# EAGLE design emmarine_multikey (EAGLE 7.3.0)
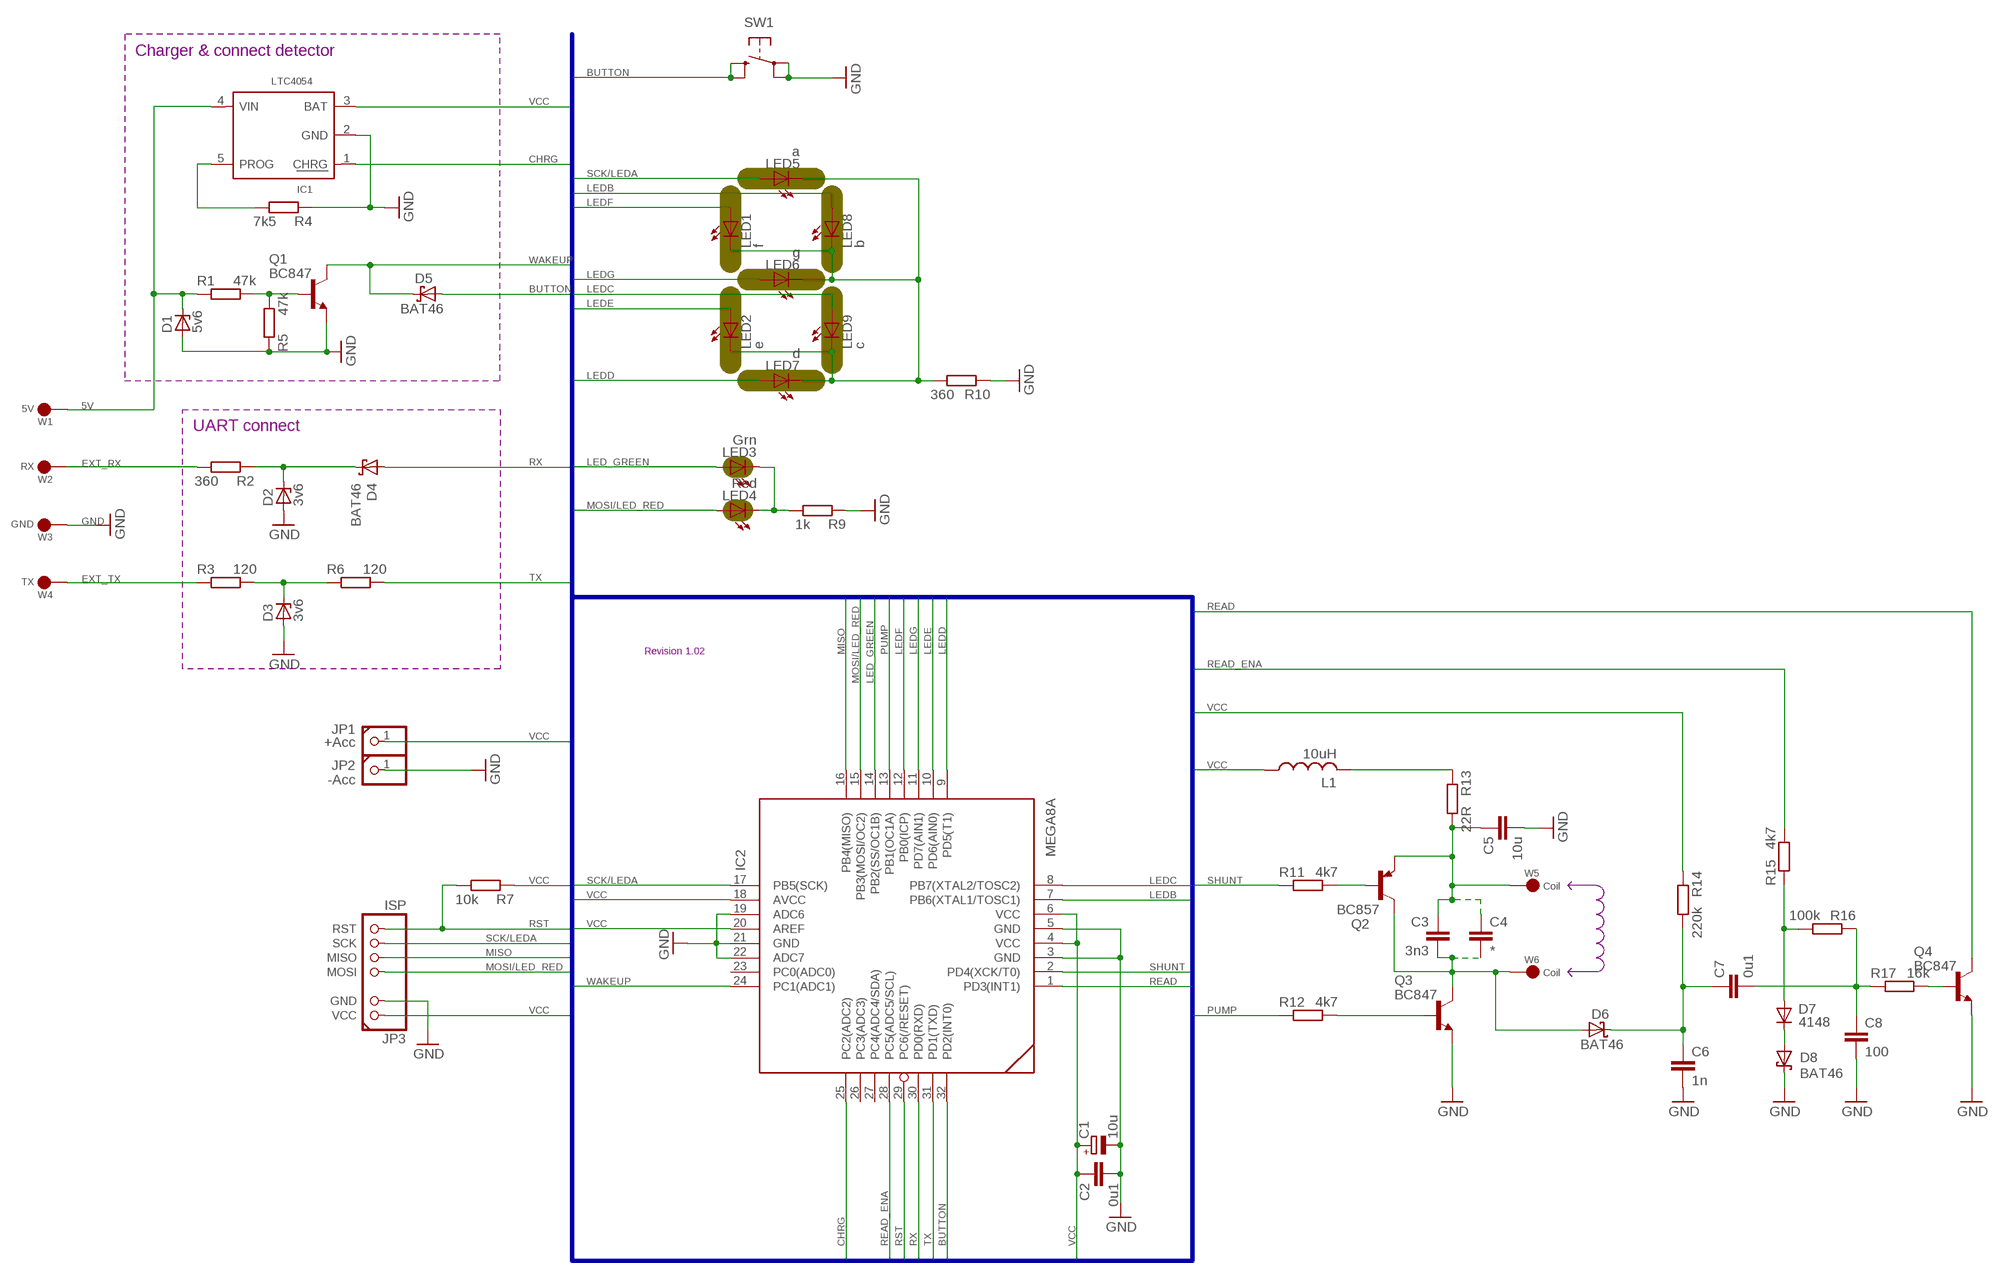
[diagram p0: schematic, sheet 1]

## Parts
C1  10u  CPOL-EUSMCA  [SMC_A]
C2  0u1  C-EUC0805T  [C0805T]
C3  3n3  C-EU050-025X075  [C050-025X075]
C4  *  C-EUC0805T  [C0805T]
C5  10u  C-EUC0805T  [C0805T]
C6  1n  C-EUC0805T  [C0805T]
C7  0u1  C-EUC0805T  [C0805T]
C8  100  C-EUC0805T  [C0805T]
D1  5v6  ZENER-DIODESOD80C  [SOD80C]
D2  3v6  ZENER-DIODESOD80C  [SOD80C]
D3  3v6  ZENER-DIODESOD80C  [SOD80C]
D4  BAT46  SCHOTTKY-DIODESOD80-R  [SOD80-R]
D5  BAT46  SCHOTTKY-DIODESOD80-R  [SOD80-R]
D6  BAT46  SCHOTTKY-DIODESOD80-R  [SOD80-R]
D7  4148  1N4148SMD  [SOD80-R]
D8  BAT46  SCHOTTKY-DIODESOD80-R  [SOD80-R]
IC1  LTC4054  [SOT23-5]
IC2  MEGA8A  MEGA8(TQFP)-AI  [TQFP32-08]
JP1  +Acc  CONN1X1/R  [1X01ROUND]
JP2  -Acc  CONN1X1/R  [1X01ROUND]
JP3  ISP  CONN1X7(2+4)_ISP+/P/NI  [1X07_ISP+POINTS_NO_INF]
L1  10uH  L-USL1210  [L1210]
LED1  f  LED0603  [CHIPLED_0603]
LED2  e  LED0603  [CHIPLED_0603]
LED3  Grn  LED0603  [CHIPLED_0603]
LED4  Red  LED0603  [CHIPLED_0603]
LED5  a  LED0603  [CHIPLED_0603]
LED6  g  LED0603  [CHIPLED_0603]
LED7  d  LED0603  [CHIPLED_0603]
LED8  b  LED0603  [CHIPLED_0603]
LED9  c  LED0603  [CHIPLED_0603]
Q1  BC847  [SOT23_THIN]
Q2  BC857  [SOT23_THIN]
Q3  BC847  [SOT23_THIN]
Q4  BC847  [SOT23_THIN]
R1  47k  R-EU_R0805T  [R0805T]
R2  360  R-EU_R0805T  [R0805T]
R3  120  R-EU_R0805T  [R0805T]
R4  7k5  R-EU_R0805T  [R0805T]
R5  47k  R-EU_R0805T  [R0805T]
R6  120  R-EU_R0805T  [R0805T]
R7  10k  R-EU_R0805T  [R0805T]
R9  1k  R-EU_R0805T  [R0805T]
R10  360  R-EU_R0805T  [R0805T]
R11  4k7  R-EU_R0805T  [R0805T]
R12  4k7  R-EU_R0805T  [R0805T]
R13  22R  R-EU_R0805T  [R0805T]
R14  220k  R-EU_R0805T  [R0805T]
R15  4k7  R-EU_R0805T  [R0805T]
R16  100k  R-EU_R0805T  [R0805T]
R17  16k  R-EU_R0805T  [R0805T]
SW1  TACT_BUTTON24.2X3.5  [BUTTON_SMD_4.2X3.5]
W1  5V  SIMPLE_WIRE/R2  [SIMPLE_WIRE_R2]
W2  RX  SIMPLE_WIRE/R2  [SIMPLE_WIRE_R2]
W3  GND  SIMPLE_WIRE/R2  [SIMPLE_WIRE_R2]
W4  TX  SIMPLE_WIRE/R2  [SIMPLE_WIRE_R2]
W5  Coil  SIMPLE_WIRE/R  [SIMPLE_WIRE_R]
W6  Coil  SIMPLE_WIRE/R  [SIMPLE_WIRE_R]

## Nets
5V: D1.C IC1.4(VIN) R1.1 W1.WIRE
BUTTON: D5.A IC2.32(PD2(INT0)) SW1.S SW1.S@1(S)
CHRG: IC1.1(CHRG) IC2.25(PC2(ADC2))
COIL: C3.2 C4.2 D6.A Q2.3(C) Q3.3(C) W6.WIRE
EXT_RX: R2.2 W2.WIRE
EXT_TX: R3.1 W4.WIRE
GND: C1.- C2.2 C5.2 C6.2 C8.2 D1.A D2.A D3.A D8.C IC1.2(GND) IC2.3(GND) IC2.5(GND) IC2.19(ADC6) IC2.21(GND) IC2.22(ADC7) JP2.1 JP3.GND Q1.2(E) Q3.2(E) Q4.2(E) R4.1 R5.1 R9.1 R10.1 SW1.P SW1.P@1(P) W3.WIRE
LED_GREEN: IC2.14(PB2(SS/OC1B)) LED3.A
LEDB: IC2.7(PB6(XTAL1/TOSC1)) LED8.A
LEDC: IC2.8(PB7(XTAL2/TOSC2)) LED9.A
LEDD: IC2.9(PD5(T1)) LED7.A
LEDE: IC2.10(PD6(AIN0)) LED2.A
LEDF: IC2.12(PB0(ICP)) LED1.A
LEDG: IC2.11(PD7(AIN1)) LED6.A
MISO: IC2.16(PB4(MISO)) JP3.MISO
MOSI/LED_RED: IC2.15(PB3(MOSI/OC2)) JP3.MOSI LED4.A
N$1: C6.1 C7.1 D6.C R14.2
N$2: D3.C R3.2 R6.1
N$3: Q2.1(B) R11.2
N$4: Q3.1(B) R12.2
N$5: Q1.1(B) R1.2 R5.2
N$6: D2.C D4.C R2.1
N$7: LED1.C LED2.C LED5.C LED6.C LED7.C LED8.C LED9.C R10.2
N$9: L1.2 R13.1
N$10: LED3.C LED4.C R9.2
N$11: C3.1 C4.1 C5.1 Q2.2(E) R13.2 W5.WIRE
N$12: IC1.5(PROG) R4.2
N$15: Q4.1(B) R17.2
N$16: C7.2 C8.1 R16.1 R17.1
N$17: D7.A R15.1 R16.2
N$18: D7.C D8.A
PUMP: IC2.13(PB1(OC1A)) R12.1
READ: IC2.1(PD3(INT1)) Q4.3(C)
READ_ENA: IC2.28(PC5(ADC5/SCL)) R15.2
RST: IC2.29(PC6(/RESET)) JP3.RST R7.2
RX: D4.A IC2.30(PD0(RXD))
SCK/LEDA: IC2.17(PB5(SCK)) JP3.SCK LED5.A
SHUNT: IC2.2(PD4(XCK/T0)) R11.1
TX: IC2.31(PD1(TXD)) R6.2
VCC: C1.+ C2.1 IC1.3(BAT) IC2.4(VCC) IC2.6(VCC) IC2.18(AVCC) IC2.20(AREF) JP1.1 JP3.+5V(VCC) L1.1 R7.1 R14.1
WAKEUP: D5.C IC2.24(PC1(ADC1)) Q1.3(C)
Unconnected: IC2.23(PC0(ADC0)) IC2.26(PC3(ADC3)) IC2.27(PC4(ADC4/SDA))

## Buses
VCC,MOSI/LED_RED,MISO,SCK/LEDA,RST,RX,RX_UP,TX,PUMP,SHUNT,READ,READ_ENA,LEDB,LEDC,LEDD,LEDE,LEDF,LEDG,LED_GREEN,BUTTON,WAKEUP,CHRG

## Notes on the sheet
- Charger & connect detector
- UART connect
- Revision 1.02

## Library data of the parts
C1 = rcl:CPOL-EU: POLARIZED CAPACITOR, European symbol
C2-C8 = rcl:C-EU: CAPACITOR, European symbol
D1-D3 = diode:ZENER-DIODE: Z-Diode
D4-D6 D8 = diode:SCHOTTKY-DIODE: Schottky Diode
D7 = diode:1N4148: DIODE
IC1 = v-reg-AL:LTC4054
IC2 = atmel:MEGA8(TQFP): MICROCONTROLLER 8 Kbytes FLASH, 1 kbytes SRAM, 512 bytes EEPROM, USART, 6-channel 10 bit ADC, 2-channel 8 bit ADC Pin compatible with Atmega48, ATMega88, ATMega168 Source: avr.lbr; MPN: ATMEGA8-16AU; OC_FARNELL: 9171371; OC_NEWARK: 73M8863
JP1 JP2 = pinhead-AL:CONN1X1
JP3 = pinhead-AL:CONN1X7(2+4)_ISP+: PIN HEADER
L1 = rcl:L-US: INDUCTOR, American symbol
LED1-LED9 = led-AL:LED
Q1 Q3 Q4 = transistor-npn-AL:BC847*: NPN Transistor
Q2 = transistor-pnp-AL:BC857*: PNP Transistror
R1-R7 R9-R17 = rcl:R-EU_: RESISTOR, European symbol
SW1 = switch-misc-AL:TACT_BUTTON2
W1-W6 = connectors-AL:SIMPLE_WIRE

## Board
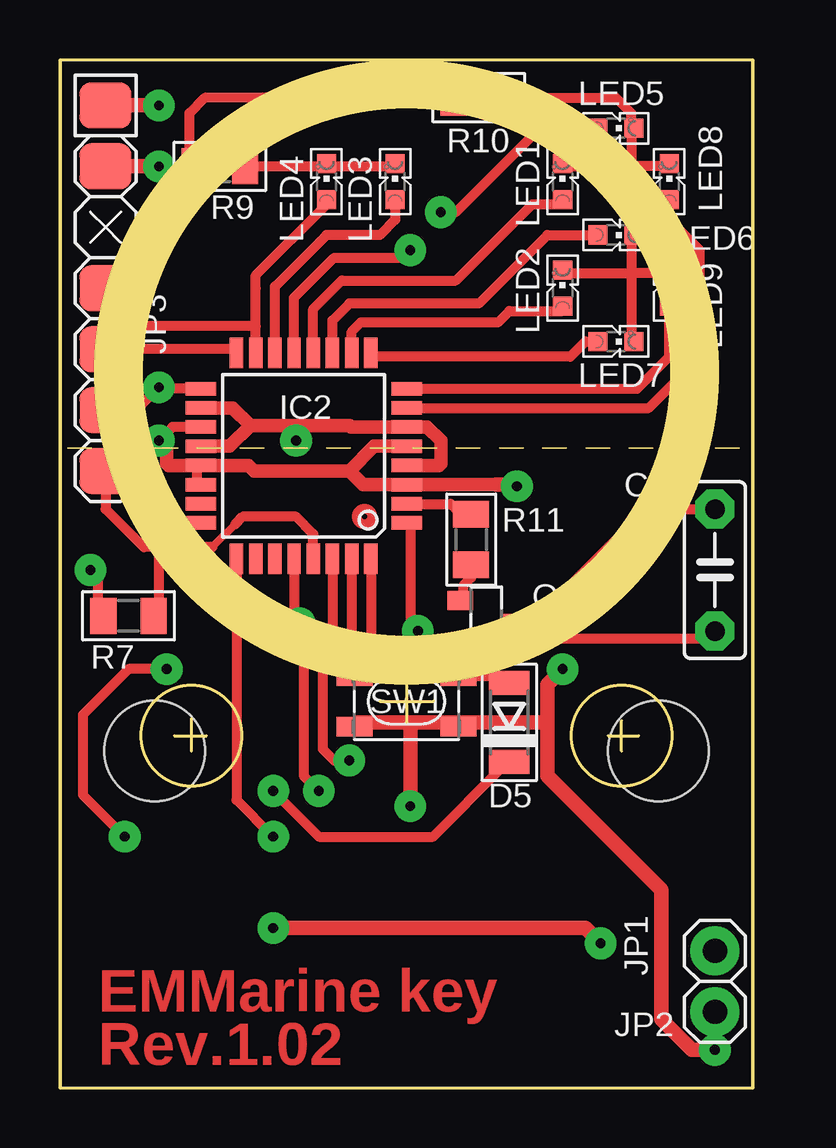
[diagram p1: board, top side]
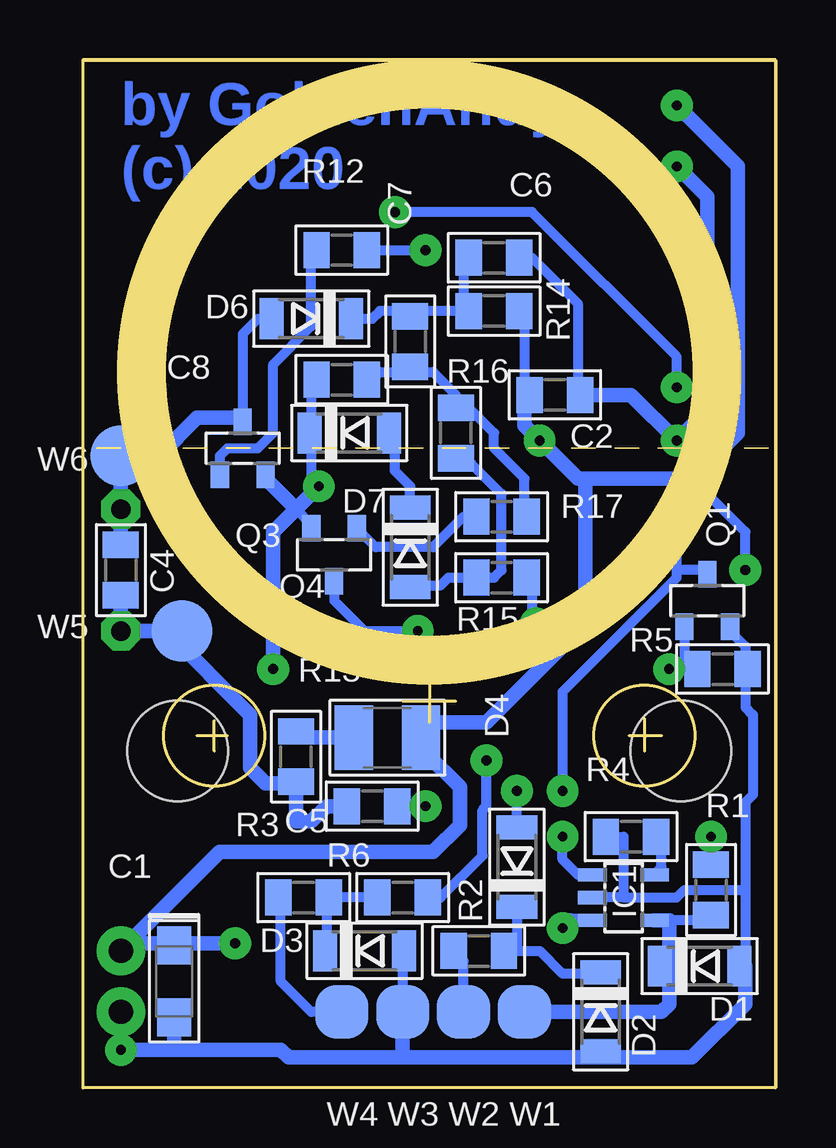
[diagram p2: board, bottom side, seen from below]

Size 28.88 x 42.85 mm. Coordinates in mm from the lower left corner, seen from the top.
Outline: 0,0 28.88,0 28.88,42.85 0,42.85 0,0
Copper layers (1*16): Top 0.035mm / dielectric 1.5mm / Bottom 0.035mm
Design rules "default": minimum track width 12mil, minimum drill 14mil, track to track 8mil, track to pad 8mil, pad to pad 8mil, via to via 8mil, smd to smd 8mil, copper to edge 20mil, drill to drill 30mil, minimum pad ring 16mil, minimum via ring 18mil, stop-mask expansion 4mil, vias tented up to drill 0mil, thermal gap 16mil
Holes 4.19 mm at 3.95,14.05 24.94,14.05
Milling: area 3.4,12.6 to 7.6,16.8; area 21.3,12.6 to 25.5,16.8; area 2.4,17.8 to 26.4,41.8; 26 lines

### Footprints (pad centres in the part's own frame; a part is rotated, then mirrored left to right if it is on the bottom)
SMC_A = smd 1.6 x 1.4: + -1.5,0; - 1.5,0
C0805T = smd 1.1 x 1.5: 1 -1.05,0; 2 1.05,0
C050-025X075 = drill 0.813 octagon: 1 -2.54,0; 2 2.54,0
SOD80C = smd 1 x 1.7: A 1.65,0; C -1.65,0
SOD80-R = smd 1 x 1.7: A 1.65,0; C -1.65,0
SOT23-5 = smd 0.55 x 1.2: 1 -0.95,-1.3; 2 0,-1.3; 3 0.95,-1.3; 4 0.95,1.3; 5 -0.95,1.3
TQFP32-08 = smd 1.27 x 0.559: 1 -4.293,2.8; 2 -4.293,2; 3 -4.293,1.2; 4 -4.293,0.4; 5 -4.293,-0.4; 6 -4.293,-1.2; 7 -4.293,-2; 8 -4.293,-2.8; 17 4.293,-2.8; 18 4.293,-2; 19 4.293,-1.2; 20 4.293,-0.4; 21 4.293,0.4; 22 4.293,1.2; 23 4.293,2; 24 4.293,2.8 | smd 0.559 x 1.27: 9 -2.8,-4.293; 10 -2,-4.293; 11 -1.2,-4.293; 12 -0.4,-4.293; 13 0.4,-4.293; 14 1.2,-4.293; 15 2,-4.293; 16 2.8,-4.293; 25 2.8,4.293; 26 2,4.293; 27 1.2,4.293; 28 0.4,4.293; 29 -0.4,4.293; 30 -1.2,4.293; 31 -2,4.293; 32 -2.8,4.293
1X01ROUND = drill 1.016 pad 2.032: 1 0,0
1X07_ISP+POINTS_NO_INF = smd 1.905 x 2.159: +5V -7.62,0; GND -5.08,0; MISO 2.54,0; MOSI 0,0; RST 7.62,0; SCK 5.08,0
L1210 = smd 1.6 x 2.7: 1 -1.4,0; 2 1.4,0
CHIPLED_0603 = smd 0.8 x 0.8: A 0,-0.75; C 0,0.75
SOT23_THIN = smd 0.8 x 1.1: 1 -0.95,-1.1; 2 0.95,-1.1; 3 0,1.1
R0805T = smd 1.1 x 1.5: 1 -1.05,0; 2 1.05,0
BUTTON_SMD_4.2X3.5 = smd 1.5 x 0.8: P -2.17,1.055; P@1 2.17,1.055; S -2.17,-1.055; S@1 2.17,-1.055
SIMPLE_WIRE_R2 = smd 2.223 x 2.223: WIRE 0,0
SIMPLE_WIRE_R = smd 2.54 x 2.54: WIRE 0,0

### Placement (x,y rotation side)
C1  25.08,4.45 270 bottom
C2  9.21,28.89 0 bottom
C3  27.3,21.59 90 top
C4  27.3,21.59 90 bottom
C5  16.83,11.75 0 bottom
C6  11.75,34.61 0 bottom
C7  15.24,31.12 270 bottom
C8  18.1,29.53 180 bottom
D1  3.18,5.08 0 bottom
D2  7.3,3.18 270 bottom
D3  17.15,5.71 0 bottom
D4  10.8,9.21 90 bottom
D5  18.73,15.24 90 top
D6  19.37,32.07 180 bottom
D7  15.24,22.54 270 bottom
D8  17.78,27.3 0 bottom
IC1  6.35,7.94 270 bottom
IC2  10.16,26.35 180 top
JP1  27.3,5.71 0 top
JP2  27.3,3.18 0 top
JP3  1.91,33.34 270 top
L1  16.19,14.61 180 bottom
LED1  20.95,37.78 0 top
LED2  20.95,33.34 0 top
LED3  13.97,37.78 0 top
LED4  11.11,37.78 0 top
LED5  23.18,40.01 270 top
LED6  23.18,35.56 270 top
LED7  23.18,31.12 270 top
LED8  25.4,37.78 0 top
LED9  25.4,33.34 0 top
Q1  2.86,20.32 0 bottom
Q2  17.78,19.37 270 top
Q3  22.23,26.67 0 bottom
Q4  18.41,22.23 180 bottom
R1  2.7,8.26 90 bottom
R2  12.38,5.71 180 bottom
R3  19.69,7.94 0 bottom
R4  6.03,10.48 0 bottom
R5  2.22,17.46 180 bottom
R6  15.56,7.94 0 bottom
R7  2.86,19.69 0 top
R9  6.67,38.42 0 top
R10  17.46,41.27 0 top
R11  17.15,22.86 270 top
R12  18.1,34.93 180 bottom
R13  20,13.81 270 bottom
R14  11.75,32.38 180 bottom
R15  11.43,21.27 0 bottom
R16  13.34,27.3 270 bottom
R17  11.43,23.81 180 bottom
SW1  14.45,16.11 180 top
W1  10.48,3.18 0 bottom
W2  13.02,3.18 0 bottom
W3  15.56,3.18 0 bottom
W4  18.1,3.18 0 bottom
W5  24.77,19.05 0 bottom
W6  27.3,26.35 0 bottom

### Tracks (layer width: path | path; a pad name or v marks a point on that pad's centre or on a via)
5V
  Bottom 0.406: R1.1 2.54,6.98 IC1.4
  Bottom 0.61: W1.WIRE 4.76,3.18 4.45,3.49 4.45,5.4 | IC1.4 4.76,6.99 | 4.76,6.99 5.08,6.98 | 4.76,6.99 4.45,6.98 4.45,5.4 | D1.C 4.45,5.4
BUTTON
  Top 0.406: IC2.32 12.96,17.41 12.7,17.15 12.68,17.17 SW1.S@1 SW1.S 16.64,17.15 18.73,17.15 D5.A
CHRG  (via drill 0.41)
  Top 0.406: v8.89,10.48 7.36,12.01 IC2.25
  Bottom 0.406: IC1.1 8.25,8.89 8.89,9.52 v8.89,10.48
COIL
  Top 0.406: Q2.3 19.69,19.37 24.45,24.13 C3.2
  Bottom 0.406: Q3.3 22.23,31.43 21.59,32.07 D6.A
  Bottom 0.61: C4.2 C3.2 W6.WIRE 25.72,26.35 24.13,27.94 22.23,27.94 Q3.3
EXT_RX
  Bottom 0.406: W2.WIRE 13.02,5.3 R2.2
EXT_TX
  Bottom 0.406: W4.WIRE 19.37,3.18 20.64,4.45 20.64,7.84 R3.1
GND  (via drill 0.41)
  Top 0.406: IC2.22 5.79,25.15 5.71,25.08 5.71,25.8 IC2.21 | 4.45,26.99 4.45,27.3 4.69,27.55 IC2.19 | 20,15.24 20.32,15.24 | SW1.P@1 12.28,15.13 12.38,15.24 | SW1.P 16.65,15.06 16.83,15.24 | R10.1 6.03,41.27 5.4,40.64 5.4,38.42 | v4.13,38.42 5.4,38.42 | R9.1 5.4,38.42
  Top 0.559: IC2.5 13.1,26.75 12.07,25.72 | 12.07,25.72 8.09,25.72 7.86,25.95 IC2.21 4.53,25.95 4.45,26.04 4.45,26.99 v4.13,26.99 | 12.07,25.72 12.63,25.15 IC2.3 18.17,25.15
  Top 0.61: JP3.GND v4.13,38.42 | v20.95,17.46 20.32,16.83 20.32,15.24 20.32,13.02 25.08,8.26 25.08,2.86 26.35,1.59 v27.3,1.59 | v14.61,11.75 14.61,15.24 | 12.38,15.24 14.61,15.24 | 14.61,15.24 16.83,15.24 20,15.24 | 18.17,25.15 18.8,25.15 v19.05,25.08
  Bottom 0.406: C6.2 10.16,34.61 8.26,32.7 8.26,28.67 C2.2 | Q4.2 19.37,23.49 20,24.13 | v19.05,25.08 19.37,25.4 19.37,27.3 D8.C 19.37,27.37 19.37,29.53 C8.2 | D3.A 15.56,5.71 W3.WIRE | 1.27,17.46 1.27,18.41 1.91,19.05 Q1.2 | 1.27,17.46 1.27,15.88 0.95,15.56 0.95,12.22 1.27,11.91 1.27,8.26 | 1.27,8.26 1.27,5.08 D1.A | R4.1 6.35,10.48 6.35,7.94 | 6.35,7.94 IC1.2 | 6.35,7.94 4.13,7.94 3.81,8.26 1.27,8.26 | R5.1 1.27,17.46
  Bottom 0.61: v4.13,38.42 2.86,37.15 2.86,28.26 v4.13,26.99 6.03,28.89 C2.2 | v19.05,25.08 20,24.13 | 20,24.13 20.95,23.18 v20.95,17.46 | JP2.1 v27.3,1.59 25.08,1.59 | Q3.2 21.27,25.4 20,24.13 | C5.2 v14.61,11.75 | C1.- 25.08,1.59 | 25.08,1.59 20.64,1.59 20.32,1.27 15.56,1.27 | 15.56,1.27 W3.WIRE | D2.A 7.3,1.27 | 7.3,1.27 15.56,1.27 | 1.27,5.08 1.27,3.49 3.49,1.27 7.3,1.27
LED_GREEN
  Top 0.406: IC2.14 8.96,33.41 11.11,35.56 13.34,35.56 13.97,36.2 LED3.A
LEDB
  Top 0.406: IC2.7 24.54,28.35 26.67,30.48 26.67,34.93 25.4,36.2 LED8.A
LEDC
  Top 0.406: IC2.8 24.07,29.15 25.4,30.48 LED9.A
LEDD
  Top 0.406: IC2.9 13.12,30.48 21.27,30.48 21.91,31.12 LED7.A
LEDE
  Top 0.406: IC2.10 12.16,31.53 12.54,31.91 18.26,31.91 18.73,32.38 20.95,32.38 LED2.A
LEDF
  Top 0.406: IC2.12 10.56,32.47 11.75,33.66 16.51,33.66 19.69,36.83 20.95,36.83 LED1.A
LEDG
  Top 0.406: IC2.11 11.36,32 12.07,32.7 17.46,32.7 20.32,35.56 LED6.A
MISO
  Top 0.406: IC2.16 7.36,30.74 7.3,30.8 JP3.MISO
MOSI/LED_RED
  Top 0.406: 8.16,31.75 3.49,31.75 JP3.MOSI | IC2.15 8.16,31.75 | LED4.A 11.11,36.83 8.16,33.88 8.16,33.34 8.16,31.75
N$1
  Bottom 0.406: C6.1 13.02,34.61 13.02,32.38 R14.2 15.24,32.38 | 15.24,32.38 16.51,32.38 16.83,32.07 D6.C | C7.1 15.24,32.38
N$2
  Bottom 0.406: R6.1 R3.2 18.73,7.94 18.73,5.78 D3.C
N$3
  Top 0.406: R11.2 17.15,21.27 16.83,20.95 16.83,20.32 Q2.1
N$4
  Bottom 0.406: Q3.1 23.18,26.36 22.86,26.67 21.59,26.67 20.95,27.3 20.95,30.16 19.37,31.75 19.37,34.93 R12.2
N$5  (via drill 0.41)
  Top 0.406: v4.45,17.46 2.86,17.46 0.95,15.56 0.95,12.22 v2.7,10.48
  Bottom 0.406: Q1.1 3.81,19.05 3.81,17.46 | 3.81,17.46 3.49,17.46 3.27,17.37 R5.2 | 3.81,17.46 v4.45,17.46 | v2.7,10.48 R1.2
N$6
  Bottom 0.406: R2.1 10.8,5.71 | D4.C 10.8,5.71 | 10.8,5.71 9.84,5.71 8.89,4.76 7.3,4.76 D2.C
N$7
  Top 0.406: R10.2 23.18,41.27 23.81,40.64 23.81,40.01 | LED5.C 23.81,40.01 | 23.81,40.01 23.81,38.42 | 23.81,38.42 23.81,35.56 | 23.81,35.56 23.81,33.97 | 23.81,33.97 23.81,31.12 LED7.C | LED6.C 23.81,35.56 | LED2.C 20.95,33.97 23.81,33.97 | LED9.C 25.4,33.97 23.81,33.97 | LED8.C 25.4,38.42 23.81,38.42 | LED1.C 20.95,38.42 23.81,38.42
N$9
  Bottom 0.406: 19.91,14.61 R13.1
  Bottom 0.61: L1.2 19.91,14.61
N$10
  Top 0.406: R9.2 11.11,38.42 | 11.11,38.42 13.97,38.42 LED3.C | LED4.C 11.11,38.42
N$11
  Top 0.406: Q2.2 16.83,18.42 16.83,18.41 17.62,18.41 17.78,18.26 19.84,18.26 20.32,18.73 26.99,18.73 C3.1
  Bottom 0.61: C5.1 18.73,11.75 19.37,11.11 20,11.11 R13.2 20.06,12.7 21.27,12.7 21.91,13.34 21.91,15.56 25.4,19.05 | W5.WIRE 25.4,19.05 | 25.4,19.05 C3.1 C4.1
N$12
  Bottom 0.406: IC1.5 4.77,9.2 4.76,9.52 4.76,10.48 R4.2
N$15
  Bottom 0.406: R17.2 13.02,23.81 14.29,22.54 16.68,22.54 Q4.1
N$16
  Bottom 0.406: R17.1 10.48,23.81 10.48,25.4 11.75,26.67 11.75,27.3 12.7,28.26 13.24,28.26 R16.1 13.34,28.89 14.29,29.84 15.24,29.84 C7.2 15.46,29.84 16.51,29.84 16.83,29.53 C8.1
N$17
  Bottom 0.406: R16.2 13.34,26.04 12.7,26.04 11.43,24.77 11.43,21.59 11.75,21.27 R15.1 13.65,21.27 13.97,20.95 15.24,20.95 D7.A
N$18
  Bottom 0.406: D7.C 15.24,25.08 15.88,25.72 15.88,27.3 D8.A
PUMP  (via drill 0.41)
  Top 0.406: IC2.13 9.76,32.94 11.43,34.61 14.29,34.61 v14.61,34.93
  Bottom 0.406: R12.1 v14.61,34.93
READ  (via drill 0.41)
  Top 0.406: IC2.1 14.55,23.55 14.61,23.5 14.61,19.37 v14.92,19.05
  Bottom 0.406: Q4.3 18.41,20.32 17.15,19.05 v14.92,19.05
READ_ENA  (via drill 0.41)
  Top 0.406: IC2.28 9.76,19.61 v10,19.37
  Bottom 0.406: R15.2 10.16,21.27 10.16,19.53 v10,19.37
RST
  Top 0.305: 7.3,23.5 6.35,22.54
  Top 0.406: IC2.29 10.56,23.09 9.84,23.81 7.62,23.81 7.3,23.5 | 6.35,22.54 4.13,22.54 | 4.13,22.54 3.49,22.54 1.91,24.13 JP3.RST | R7.2 4.13,19.69 4.13,22.54
RX  (via drill 0.41)
  Top 0.406: IC2.30 11.36,19.06 10.16,17.86 10.16,13.02 v10.8,12.38
  Bottom 0.406: D4.A v10.8,12.38
SCK/LEDA  (via drill 0.41)
  Top 0.406: IC2.17 4.19,29.15 v4.13,29.21 3.18,28.26 JP3.SCK | v15.88,36.51 16.51,36.51 20,40.01 LED5.A
  Bottom 0.406: v4.13,29.21 4.13,30.48 10.16,36.51 v15.88,36.51
SHUNT
  Top 0.406: R11.1 17.15,24.13 16.51,24.13 16.29,24.35 IC2.2
TX  (via drill 0.41)
  Top 0.406: IC2.31 12.16,18.91 10.95,17.7 10.95,14.13 11.43,13.65 v12.07,13.65
  Bottom 0.406: R6.2 13.97,7.94 12.22,9.68 12.22,11.59 12.07,11.75 v12.07,13.65
VCC  (via drill 0.41)
  Top 0.406: R7.1 1.59,19.69 1.59,21.27 v1.27,21.59
  Top 0.559: IC2.4 15.79,25.95 15.88,26.04 15.88,26.99 15.31,27.55 IC2.6 12.13,27.55 12.07,27.62 9.84,27.62 | IC2.20 7.07,26.75 7.94,27.62 | IC2.18 7.21,28.35 7.94,27.62 | 7.94,27.62 9.84,27.62 | v9.84,26.99 9.84,27.62
  Top 0.61: JP3.+5V v4.13,40.96 | v8.89,6.67 21.91,6.67 v22.54,6.03
  Bottom 0.406: C2.1 10.48,28.58 | R14.1 10.48,32.38 10.48,27.94 | v1.27,21.59 1.27,23.18 3.49,25.4
  Bottom 0.559: IC1.3 7.94,6.99 8.57,6.98
  Bottom 0.61: v4.13,40.96 1.59,38.42 1.59,27.3 3.49,25.4 7.94,25.4 | 7.94,25.4 8.26,25.4 v9.84,26.99 10.48,27.62 10.48,27.94 10.48,28.58 | 14.61,14.61 L1.1 | 14.61,14.61 14.61,13.97 13.18,12.54 13.18,10.95 14.29,9.84 23.18,9.84 JP1.1 26.99,6.03 25.08,6.03 C1.+ 25,6.03 v22.54,6.03 | 14.61,14.61 14.61,15.24 12.07,15.24 7.94,19.37 7.94,25.4 | 8.57,6.98 v8.89,6.67
WAKEUP  (via drill 0.41)
  Top 0.406: IC2.24 4.39,23.55 v4.13,23.81 | v8.89,12.38 10.8,10.48 15.56,10.48 18.41,13.34 18.73,13.34 D5.C
  Bottom 0.406: v8.89,12.38 8.89,16.51 4.13,21.27 4.13,21.59 | Q1.3 2.86,21.59 4.13,21.59 | 4.13,21.59 v4.13,23.81
(copper drawn outside any net)
  shapes: Top circle x1

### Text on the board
Top: EMMarine key | Rev.1.02
Bottom: by GoldenAndy / (c) 2020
